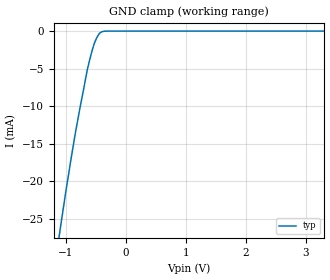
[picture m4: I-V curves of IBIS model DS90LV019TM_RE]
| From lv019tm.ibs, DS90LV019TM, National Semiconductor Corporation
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|   RECEIVER Enable MODEL {START}
[Model]   DS90LV019TM_RE
Model_type   Input
|Signals   RE
Vinh = 2.0
Vinl = 0.8
|   typ   min   max
C_comp   3.83pF   NA   NA
|   typ   min   max
[Temperature Range]   25.0   NA   NA
[Voltage range]   3.3V   3.0V   3.6V
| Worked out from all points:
|   GND clamp passes 1 mA (typ) near -0.49 V on its own axis
[GND_clamp]
|Voltage   I(typ)   I(min)   I(max)
-3.3V     -150mA     NA         NA
-1.102V   -26.83mA   NA         NA
-1.072V   -25.18mA   NA         NA
-1.011V   -21.95mA   NA         NA
-919mV    -17.32mA   NA         NA
-828mV    -12.99mA   NA         NA
-644mV    -5.219mA   NA         NA
-582mV    -3.185mA   NA         NA
-521mV    -1.553mA   NA         NA
-460mV    -532uA     NA         NA
-398mV    -83.34uA   NA         NA
3.3V      1.048uA    NA         NA
[Power_clamp]
| Note that the[POWER_clamp]voltage table is referenced to Vcc
| and is calculated using Vtable=Vcc - Vmeasured.
|   Voltage   I(typ)   I(min)   I(max)
-3.3V     0A         NA         NA
0V        0A         NA         NA
